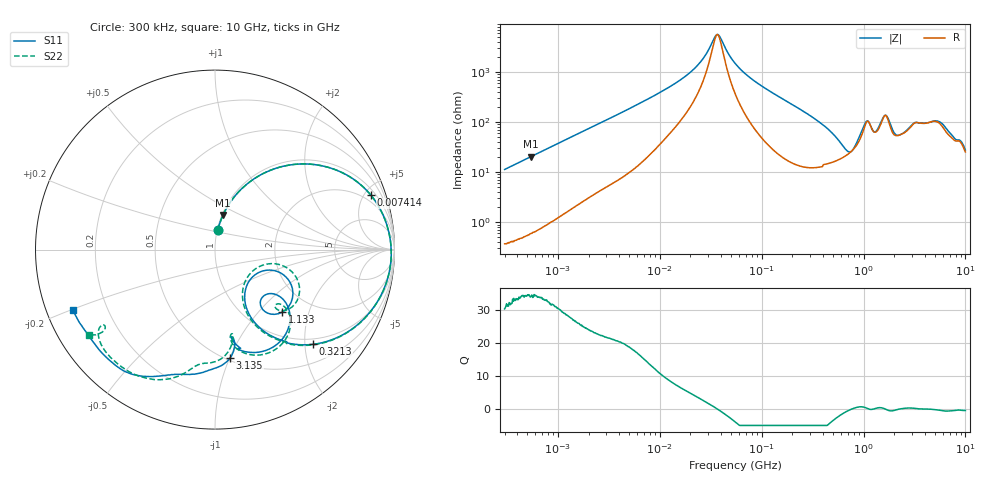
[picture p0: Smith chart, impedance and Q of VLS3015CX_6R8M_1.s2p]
! S-Parameter Data Generated by TDK Corporation
! Copyright(C) 2020 TDK Corporation.
! All Rights Reserved.
! TDK P/N: VLS3015CX-6R8M-1 (Inductor)
! Property: L=6.8uH at 1MHz
! Size(LxWxT): 3x3x1.5mm
! Model Type: s2p (Touchstone File Format Version 1.0)
! Frequency: DC=Yes Start=0.3MHz Stop=10000MHz 802points Log-sweep
! Model Generated on Aug. 18, 2020
! Port Assignments:
!  1 ---@@@--- 2
! Applicable Conditions:
!  Temperature = 25 degC
!  DC Bias Current = 0 A
!  Small Signal Operation
! Terms and conditions regarding TDK Simulation Models
! (1)This simulation model is being provided solely for informational purposes. Please refer to the specifications of the products in terms of detailed characteristics of such products.
! (2)In no event shall TDK Corporation of any of its subsidiaries be liable for any loss or damage arising, directly or indirectly,
!  From any information contained in this simulation model, including, but not limited to loss or damages arising from any inaccuracies, omissions or errors in connection with such information.
! (3)Any and all copyrights on this simulation model are owned by TDK Corporation.
!  Duplication or redistribution of this simulation model without prior written permission from TDK Corporation is prohibited.
! (4)This simulation model is subject to any modification or change without any prior notice.
! (5)Neither TDK Corporation nor any of its subsidiaries shall make any warranty, express or implied,
!  Including but not limited to the correctness, implied warranties of merchantability and fitness for a particular purpose with respect to this simulation models.
! (6)The use of this simulation model shall be deemed to have consented to the terms and conditions hereof.
# Hz S MA R 50
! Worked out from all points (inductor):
!   801 points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, 300 kHz to 10 GHz, reference 50 ohm
!   read as one part in series: L = 5.97 uH near 318.3 kHz
!   highest Q = 34.6 at 542.3 kHz (marker M1), where L = 5.96 uH
!   self-resonance near 36.73 MHz
!   S11 on the Smith chart (normalised r, x): 300 kHz: 1.01, +0.23; 7.414 MHz: 1.41, +5.58; 321.3 MHz: 0.87, -2.17; 1.133 GHz: 1.44, -1.36; 3.135 GHz: 0.52, -1.00; 10 GHz: 0.08, -0.20
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300000  0.112 81.8  0.9898 -6.4  0.99 -6.4  0.1119 81.8
542347  0.198 76.9  0.9744 -11.4  0.9743 -11.4  0.1979 76.9
1713600  0.5253 56.0  0.8305 -31.7  0.8304 -31.7  0.5254 56.0
7413963  0.9206 19.2  0.332 -66.9  0.3319 -66.9  0.9206 19.2
9671944  0.9448 14.4  0.2541 -70.5  0.2541 -70.5  0.9448 14.4
2.220835e7  0.9769 3.9  0.08154 -72.0  0.08153 -72.0  0.9769 3.9
3.642588e7  0.9822 -0.9  0.01771 -5.1  0.0177 -5.1  0.9822 -0.9
5.477226e7  0.9814 -5.1  0.0659 70.4  0.06589 70.4  0.9814 -5.2
1.540638e8  0.9326 -21.7  0.3029 64.3  0.3029 64.3  0.9326 -21.9
3.126428e8  0.769 -43.1  0.5731 41.5  0.573 41.4  0.7686 -43.5
3.212744e8  0.7582 -44.1  0.5845 40.2  0.5844 40.2  0.7577 -44.5
5.580434e8  0.4506 -61.7  0.7669 10.4  0.7668 10.4  0.4466 -62.7
7.956093e8  0.2578 -40.3  0.7661 -15.4  0.766 -15.4  0.2373 -40.1
9.560117e8  0.3785 -19.4  0.6338 -31.2  0.6336 -31.2  0.3598 -13.1
1.133369e9  0.5115 -43.0  0.4787 -21.6  0.4787 -21.6  0.5388 -34.3
1.418928e9  0.4138 -36.8  0.5384 -37.8  0.5384 -37.8  0.49 -39.4
1.767019e9  0.6314 -61.2  0.4101 -22.8  0.4102 -22.8  0.6447 -64.6
2.112126e9  0.5409 -77.5  0.5455 -33.1  0.5455 -33.1  0.5004 -80.2
3.135132e9  0.6088 -82.0  0.3815 -65.1  0.3814 -65.1  0.5996 -85.5
5.849356e9  0.8261 -122.2  0.2115 -72.6  0.2114 -72.7  0.8176 -119.6
8.322921e9  0.8516 -142.3  0.1876 -83.6  0.1872 -83.8  0.7579 -146.3
1e10  0.86 -157.1  0.1829 -83.8  0.1821 -83.8  0.8456 -145.8
